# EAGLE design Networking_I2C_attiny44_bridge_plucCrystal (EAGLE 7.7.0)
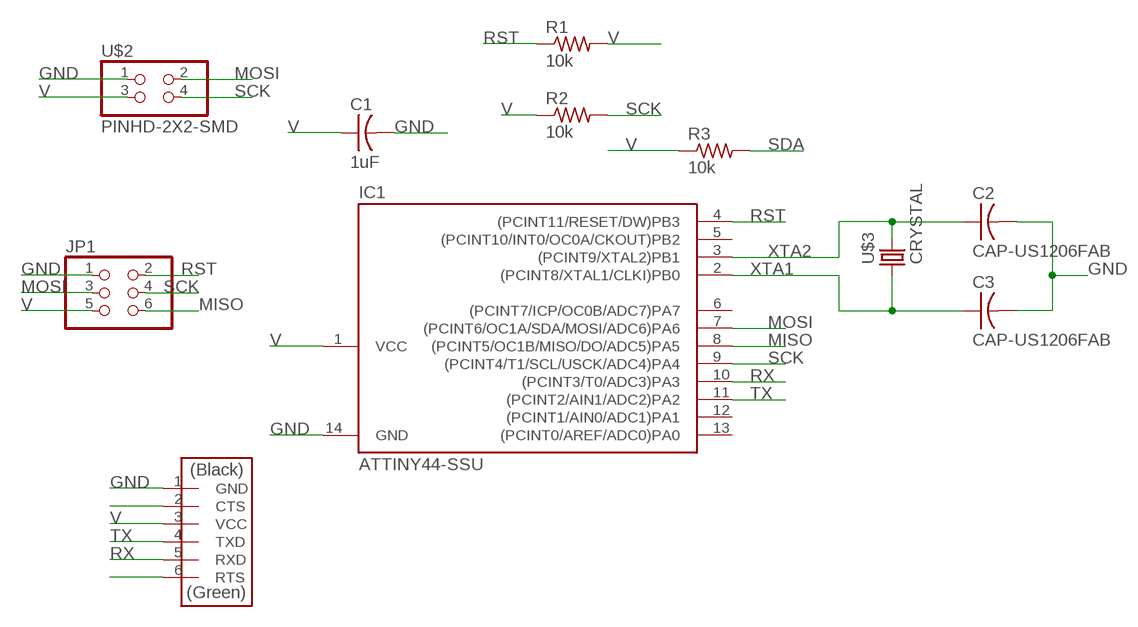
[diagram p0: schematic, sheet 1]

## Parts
C1  1uF  CAP-US1206FAB  [C1206FAB]
C2  CAP-US1206FAB  [C1206FAB]
C3  CAP-US1206FAB  [C1206FAB]
IC1  ATTINY44-SSU  [SOIC14]
JP1  PINHD-2X3-SMD  [2X03SMD]
R1  10k  RES-US1206FAB  [R1206FAB]
R2  10k  RES-US1206FAB  [R1206FAB]
R3  10k  RES-US1206FAB  [R1206FAB]
U$1  FTDI-SMD-HEADER  [1X06SMD]
U$2  PINHD-2X2-SMD  [2X02SMD]
U$3  CRYSTAL  [2-SMD-5X3MM]

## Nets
GND: C1.2 C2.2 C3.2 IC1.14(GND) JP1.1 U$1.1(GND) U$2.1
MISO: IC1.8((PCINT5/OC1B/MISO/DO/ADC5)PA5) JP1.6
MOSI: IC1.7((PCINT6/OC1A/SDA/MOSI/ADC6)PA6) JP1.3 U$2.2
N$2: U$1.2(CTS)
N$6: U$1.6(RTS)
RST: IC1.4((PCINT11/RESET/DW)PB3) JP1.2 R1.1
RX: IC1.10((PCINT3/T0/ADC3)PA3) U$1.5(RXD)
SCK: IC1.9((PCINT4/T1/SCL/USCK/ADC4)PA4) JP1.4 R2.2 U$2.4
SDA: R3.2
TX: IC1.11((PCINT2/AIN1/ADC2)PA2) U$1.4(TXD)
V: C1.1 IC1.1(VCC) JP1.5 R1.2 R2.1 R3.1 U$1.3(VCC) U$2.3
XTA1: C3.1 IC1.2((PCINT8/XTAL1/CLKI)PB0) U$3.P$1
XTA2: C2.1 IC1.3((PCINT9/XTAL2)PB1) U$3.P$2
Unconnected: IC1.5((PCINT10/INT0/OC0A/CKOUT)PB2) IC1.6((PCINT7/ICP/OC0B/ADC7)PA7) IC1.12((PCINT1/AIN0/ADC1)PA1) IC1.13((PCINT0/AREF/ADC0)PA0)

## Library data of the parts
C1-C3 = fab:CAP-US
IC1 = fab:ATTINY44
JP1 = fab:PINHD-2X3-SMD: PIN HEADER
R1-R3 = fab:RES-US: Resistor (US Symbol)
U$1 = fab:FTDI-SMD-HEADER
U$2 = fab:PINHD-2X2-SMD
U$3 = fab:CRYSTAL

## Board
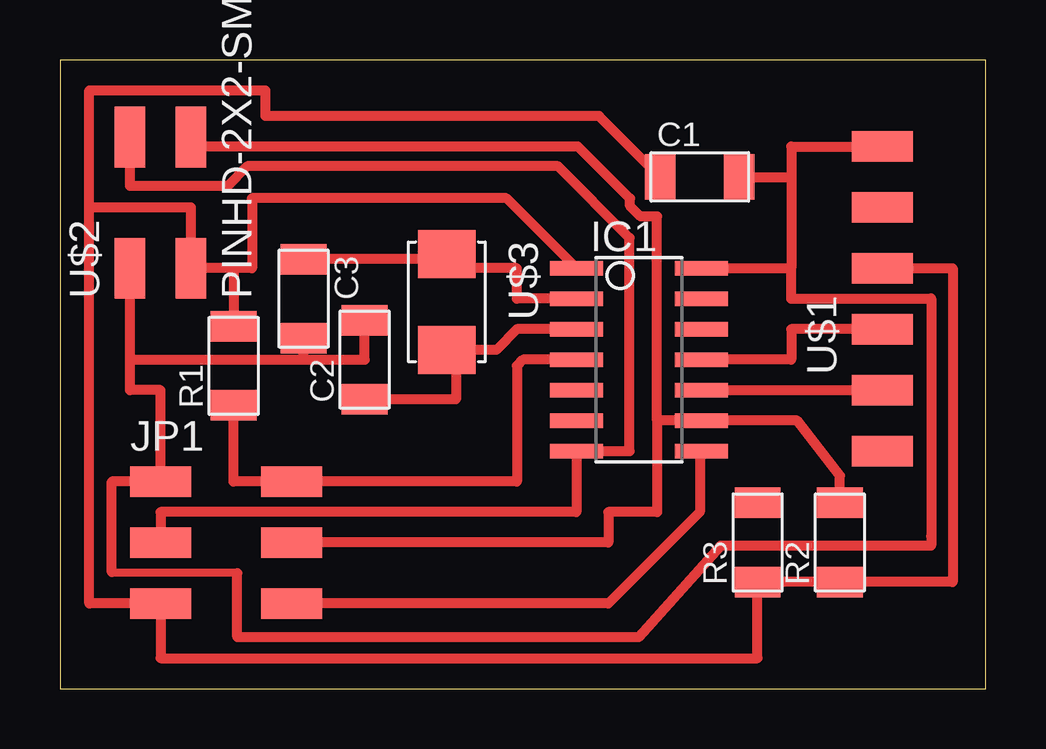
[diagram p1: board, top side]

Size 38.59 x 26.21 mm. Coordinates in mm from the lower left corner, seen from the top.
Outline: 0,0 38.59,0 38.59,26.21 0,26.21 0,0
Copper layers (1*16): Top 0.035mm / dielectric 1.5mm / Bottom 0.035mm
Design rules "default *": minimum track width 6mil, minimum drill 0.35mm, track to track 0.42mm, track to pad 0.42mm, pad to pad 0.42mm, via to via 0.42mm, smd to smd 0.42mm, copper to edge 40mil, drill to drill 6mil, minimum pad ring 10mil, minimum via ring 8mil, stop-mask expansion 4mil, vias tented up to drill 0mil, thermal gap 10mil

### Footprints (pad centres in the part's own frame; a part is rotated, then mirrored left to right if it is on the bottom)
C1206FAB = smd 1.27 x 1.905: 1 -1.651,0; 2 1.651,0
SOIC14 = smd 0.61 x 2.21: 1 -3.81,-2.603; 2 -2.54,-2.603; 3 -1.27,-2.603; 4 0,-2.603; 5 1.27,-2.603; 6 2.54,-2.603; 7 3.81,-2.603; 8 3.81,2.603; 9 2.54,2.603; 10 1.27,2.603; 11 0,2.603; 12 -1.27,2.603; 13 -2.54,2.603; 14 -3.81,2.603
2X03SMD = smd 2.54 x 1.27: 1 -2.54,2.54; 2 2.92,2.54; 3 -2.54,0; 4 2.92,0; 5 -2.54,-2.54; 6 2.92,-2.54
R1206FAB = smd 1.27 x 1.905: 1 -1.651,0; 2 1.651,0
1X06SMD = smd 2.54 x 1.27: 1 0,6.35; 2 0,3.81; 3 0,1.27; 4 0,-1.27; 5 0,-3.81; 6 0,-6.35
2X02SMD = smd 2.54 x 1.27: 1 -2.54,1.27; 2 2.92,1.27; 3 -2.54,-1.27; 4 2.92,-1.27
2-SMD-5X3MM = smd 2 x 2.4: P$1 -2,0; P$2 2,0

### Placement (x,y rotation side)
C1  26.67,21.34 0 top
C2  12.7,13.72 90 top
C3  10.16,16.26 270 top
IC1  24.13,13.72 270 top
JP1  6.73,6.1 0 top
R1  7.24,13.46 90 top
R2  32.51,6.1 90 top
R3  29.08,6.1 90 top
U$1  34.29,16.26 0 top
U$2  4.19,20.07 90 top
U$3  16.13,16.13 270 top

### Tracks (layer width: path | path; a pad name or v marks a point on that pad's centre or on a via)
GND
  Top 0.35: 7.39,4.83 2.16,4.85
  Top 0.406: C1.2 30.48,21.34 | U$1.1 30.48,22.61 30.48,21.34 | 2.92,13.72 2.92,12.45 4.19,12.45 JP1.1 2.16,8.64 2.16,4.85 | 2.92,13.72 U$2.1 | 7.39,4.83 7.39,2.16 24.13,2.16 27.54,5.97 36.32,5.97 36.32,5.99 36.32,6.35 36.32,16.27 30.48,16.27 | IC1.14 30.48,17.53 | 30.48,21.34 30.48,17.53 | 2.92,13.72 10.16,13.72 | 10.16,13.72 C3.2 | 10.16,13.72 12.7,13.72 C2.2 | 30.48,16.27 30.48,17.53 | 30.48,16.27 30.48,16.26
MISO
  Top 0.406: IC1.8 26.67,9.84 26.67,7.37 22.86,3.56 JP1.6
MOSI
  Top 0.406: JP1.3 4.19,7.37 21.53,7.37 IC1.7 23.75,9.91 23.75,18.8 20.77,21.78 7.81,21.78 6.99,20.95 2.92,20.95 U$2.2
RST
  Top 0.406: IC1.4 19.3,13.72 19.05,13.46 19.05,8.64 JP1.2 7.24,8.64 R1.1
RX
  Top 0.406: IC1.10 U$1.5
SCK
  Top 0.406: 24.89,11.18 IC1.9 30.73,11.18 32.51,8.89 R2.2 | JP1.4 22.86,6.1 22.86,7.37 24.89,7.37 24.89,11.18 | 24.89,11.18 24.89,19.68 24.2,19.68 23.76,20.12 23.76,20.43 21.59,22.61 5.46,22.61 U$2.4
TX
  Top 0.406: U$1.4 30.48,14.99 30.48,13.72 IC1.11
V
  Top 0.406: IC1.1 18.61,20.45 8,20.45 8,17.53 7.24,17.53 | 7.24,17.53 R1.2 | U$1.3 37.21,17.53 37.21,4.45 R2.1 R3.1 29.08,1.27 4.19,1.27 JP1.5 1.22,3.56 1.22,20.07 | C1.1 22.48,23.88 8.56,23.88 8.56,24.94 1.22,24.94 1.22,20.07 | 7.24,17.53 U$2.3 5.46,20.07 1.22,20.07
XTA1
  Top 0.406: IC1.2 19.05,16.26 19.05,17.53 16.73,17.53 U$3.P$1 15.91,17.91 C3.1
XTA2
  Top 0.406: IC1.3 19.05,14.99 18.19,14.13 U$3.P$2 16.51,13.75 16.51,12.06 C2.1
